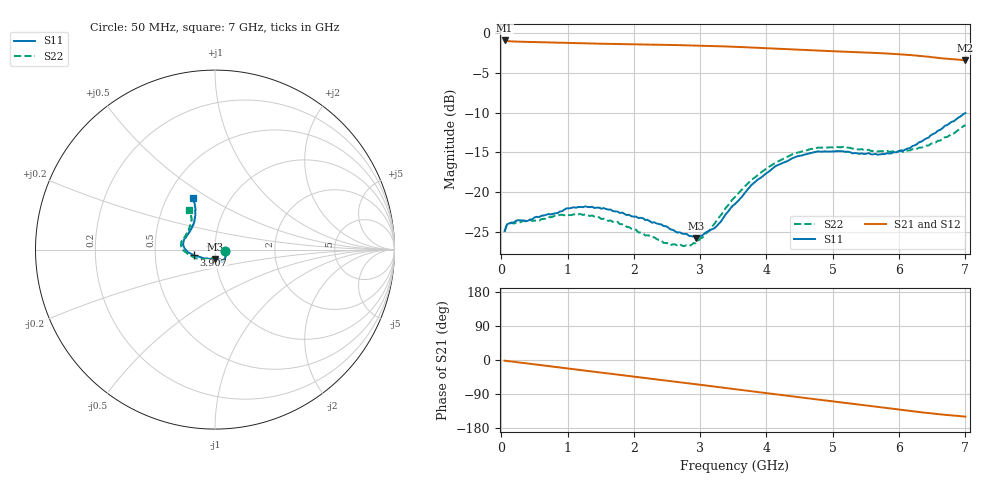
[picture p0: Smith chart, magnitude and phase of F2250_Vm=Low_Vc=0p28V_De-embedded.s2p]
! Integrated Device Technology
! Corporate Headquarters
! 6024 Silver Creek Valley Road
! San Jose, CA 95138  USA
! Phone:  1-408-284-8200
! Toll Free:  1-800-223-1366
! Webpage:  http://www.idt.com/
! Timing and RF Division
! 515 Groton Road, Suite 102
! Westford, MA 01886-6024
! Device:  F2250
! Description: Voltage Variable RF Attenuator
! Frequency:  50.0 -  6000.00 MHz
! Package:  3x3 mm Thin QFN Plastic Package: 16 pin
! Ports:  2 RF, 3 DC
!  Pin  1  = GND
!  Pin  2  = NC
!  Pin  3  = RF1  = Port 1
!  Pin  4  = NC
!  Pin  5  = GND
!  Pin  6  = GND
!  Pin  7  = GND
!  Pin  8  = GND
!  Pin  9  = NC
!  Pin 10  = RF2  = Port 2
!  Pin 11  = NC
!  Pin 12  = GND
!  Pin 13  = GND
!  Pin 14  = VCNTRL
!  Pin 15  = VDD
!  Pin 16  = VMODE
! Vcntrl:  0.280 Volts
! Vmode:  +0.000 Volts
! Vdd:  +3.30  Volts
! Current:  1.112 mA
! Data:  The device was measured on a the F2250 evaluation board which has
!  individual transmission lines to the RF pins.  Data was collected
!  using a calibrated network analyzer.  The evaluation board was
!  de-embedded using a TRL calibration technique.
!  The reference plane is the edge of the package pin.
! Misc:  SN 10
!  Action Tracker AT0258
! Date Measured:  2014-11-26
! Date:  2015-10-15  MJV
! Note:
!  Integrated Device Technology supplies this data as a sample of measured
!  data at the package pin for this product.  Your particular data for this
!  product may vary.
!  Data was taken at 25 degrees C.
!  Integrated Device Technology reserves the right to change this data at anytime.
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# GHz S dB R 50
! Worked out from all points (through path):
!   201 points, 50 MHz to 7 GHz, reference 50 ohm
!   highest |S21| = -0.94 dB at 50 MHz (marker M1); lowest = -3.4 dB at 7 GHz (marker M2)
!   group delay of S21, straight-line fit = 60 ps
!   lowest |S11| = -25.7 dB at 2.934 GHz (marker M3), VSWR 1.11, Z = 49.7 - j5.15 ohm
!   |S11| at or under -10 dB: start of sweep to end of sweep
!   |S22| runs from -26.8 to -11.6 dB; largest |S21 - S12| = 0.00032
!   S11 on the Smith chart (normalised r, x): 50 MHz: 1.12, -0.02; 3.907 GHz: 0.79, -0.05; 7 GHz: 0.67, +0.43
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0.05  -24.85 -9.5  -0.94 -1.8  -0.94 -1.8  -24.96 -9.9
0.08475  -24.03 -9.4  -1.01 -2.5  -1.01 -2.5  -24.09 -9.2
0.15425  -23.81 -11.6  -1.06 -4.0  -1.06 -4.0  -23.85 -10.9
0.57125  -23.12 -29.5  -1.16 -13.1  -1.16 -13.1  -23.57 -30.1
0.884  -22.42 -45.1  -1.22 -19.9  -1.22 -19.9  -22.84 -46.4
1.2315  -21.88 -55.2  -1.30 -27.4  -1.30 -27.4  -22.84 -59.3
1.75275  -22.43 -61.9  -1.39 -38.4  -1.39 -38.4  -23.71 -66.4
2.37825  -24.01 -62.8  -1.48 -51.8  -1.48 -51.8  -25.99 -68.1
2.552  -24.67 -67.0  -1.51 -55.6  -1.51 -55.6  -26.64 -73.7
2.83  -25.47 -82.0  -1.56 -61.7  -1.56 -61.7  -26.76 -92.8
2.93425  -25.73 -90.9  -1.58 -64.0  -1.58 -64.0  -26.39 -101.5
3.21225  -24.53 -120.4  -1.64 -70.2  -1.64 -70.2  -23.97 -127.2
3.525  -21.49 -147.1  -1.74 -77.1  -1.74 -77.1  -20.60 -146.1
3.76825  -19.14 -160.4  -1.83 -82.5  -1.83 -82.5  -18.48 -156.5
3.90725  -18.22 -164.8  -1.88 -85.5  -1.89 -85.5  -17.59 -162.6
4.1505  -16.66 -173.1  -1.98 -90.8  -1.98 -90.8  -16.22 -171.2
4.7065  -15.01 172.7  -2.19 -102.8  -2.19 -102.8  -14.55 175.8
5.15825  -14.87 162.0  -2.35 -112.6  -2.35 -112.6  -14.31 166.6
5.85325  -15.14 138.8  -2.60 -127.5  -2.60 -127.5  -14.93 151.5
6.166  -14.45 127.9  -2.77 -134.3  -2.77 -134.3  -14.75 142.7
6.444  -13.15 119.6  -2.98 -140.1  -2.98 -140.1  -14.14 133.3
7  -10.05 113.2  -3.42 -149.4  -3.42 -149.4  -11.57 123.8
